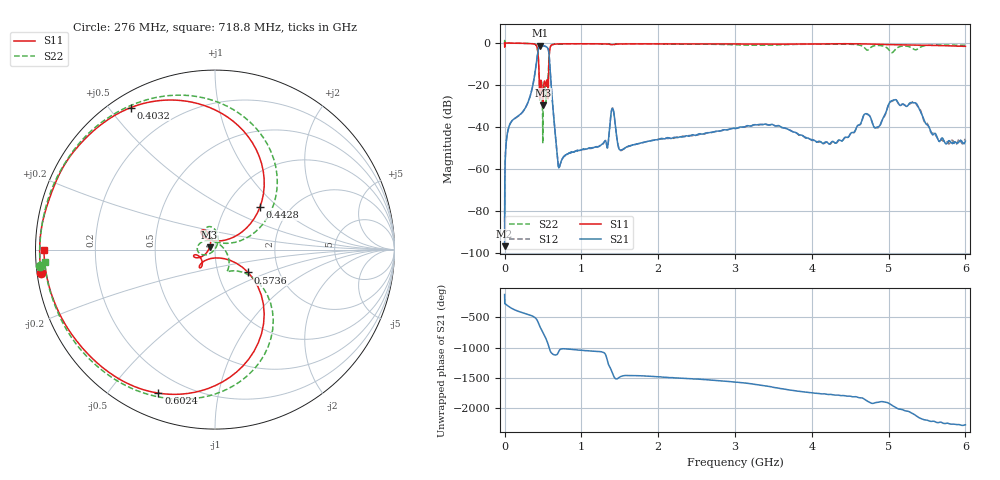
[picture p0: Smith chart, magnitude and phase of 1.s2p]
#  HZ  S  DB  R  50.00
! Rohde & Schwarz Vector Network Analyzer
! Rohde-Schwarz,ZNL6-2Port,1323001206101378,1.50.1.34-21.10.1.104
! Created: UTC 4/19/2023, 7:14:21 AM
! freq[Hz]  db:S11  ang:S11  db:S21  ang:S21  db:S12  ang:S12  db:S22  ang:S22
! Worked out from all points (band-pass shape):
!   5001 points, 5 kHz to 6 GHz, reference 50 ohm
!   highest |S21| = -1.19 dB at 460.8 MHz (marker M1); lowest = -97.0 dB at 5 kHz (marker M2)
!   |S21| within 3 dB of the highest: 431.7 MHz to 574.7 MHz (143 MHz wide, 28.4 % of centre)
!   lowest |S11| = -29.7 dB at 495.6 MHz (marker M3), VSWR 1.07, Z = 47 + j1.12 ohm
!   |S11| at or under -10 dB: 443.8 MHz to 576 MHz (132.2 MHz wide, 25.9 % of centre)
!   |S22| runs from -47.9 to 1.2 dB; largest |S21 - S12| = 0.023
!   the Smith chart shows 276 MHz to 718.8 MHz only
!   S11 on the Smith chart (normalised r, x): 276 MHz: 0.01, -0.07; 403.2 MHz: 0.06, +0.57; 442.8 MHz: 1.43, +0.77; 573.6 MHz: 1.39, -0.37; 602.4 MHz: 0.11, -0.68; 718.8 MHz: 0.02, +0.00
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5000  0.00 0.0  -96.96 -124.7  -85.36 121.6  -0.01 -0.0
5.760495e7  -0.02 -56.6  -39.77 34.6  -39.85 33.1  -0.05 -56.6
1.620049e8  -0.06 -125.9  -35.21 -33.9  -35.29 -35.1  -0.12 -126.6
2.760048e8  -0.19 -172.4  -30.59 -80.4  -30.63 -82.2  -0.20 -174.5
4.032047e8  -0.73 120.7  -12.30 -154.0  -12.32 -153.7  -0.78 113.2
4.428046e8  -9.23 43.5  -2.02 116.6  -2.01 117.8  -9.28 31.4
4.608046e8  -22.91 125.3  -1.19 62.5  -1.17 64.0  -22.83 115.6
4.956046e8  -29.73 158.6  -1.22 -23.3  -1.21 -22.1  -37.71 65.8
5.244046e8  -18.35 -165.3  -1.52 -95.0  -1.51 -93.8  -20.84 157.2
5.736045e8  -12.99 -34.6  -3.92 101.1  -3.92 102.2  -10.14 -37.3
6.024045e8  -1.31 -111.5  -18.10 2.9  -18.08 4.7  -1.27 -105.7
7.188044e8  -0.42 180.0  -58.47 44.1  -58.55 43.2  -0.43 -175.7
1.000804e9  -0.36 135.0  -51.00 35.3  -50.89 35.2  -0.36 137.2
1.326004e9  -0.46 102.2  -48.18 -77.3  -48.05 -79.0  -0.46 103.3
1.405204e9  -0.75 96.5  -31.22 14.1  -31.03 11.9  -0.93 97.5
1.512004e9  -0.41 88.4  -51.07 -38.4  -51.31 -40.4  -0.41 89.7
2.000403e9  -0.40 50.9  -46.09 -42.4  -45.87 -43.3  -0.41 51.4
3.000002e9  -0.44 -17.4  -40.72 -131.4  -40.82 -130.5  -0.83 -19.0
4.000802e9  -0.48 -84.8  -46.14 53.3  -46.44 52.1  -0.58 -88.4
4.856401e9  -0.59 -149.0  -40.07 -104.8  -40.48 -104.6  -1.13 -155.4
5.000401e9  -0.76 -160.1  -29.39 -118.8  -29.09 -118.3  -3.09 -175.8
6e9  -1.58 118.6  -46.81 -116.1  -45.86 -122.7  -1.10 117.8
